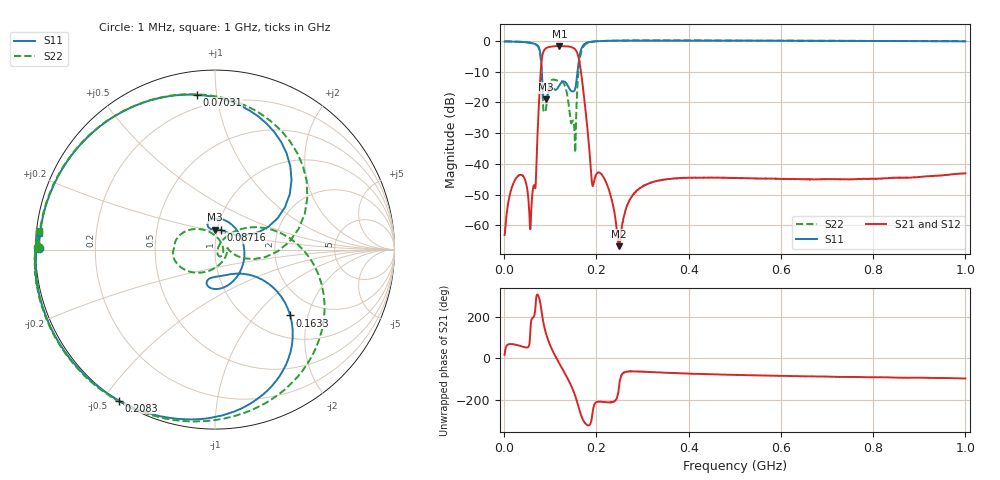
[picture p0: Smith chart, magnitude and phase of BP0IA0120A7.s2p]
!Agilent Technologies,E8358A,US41080443,A.07.50.56
!Agilent E8358A: A.07.50.56
!Date: Tuesday, October 31, 2017 22:11:44
!Correction: S11(Full 2 Port(1,2))
!S21(Full 2 Port(1,2))
!S12(Full 2 Port(1,2))
!S22(Full 2 Port(1,2))
!S2P File: Measurements: S11, S21, S12, S22:
# Hz S  dB  R 50
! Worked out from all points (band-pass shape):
!   1601 points, 1 MHz to 1 GHz, reference 50 ohm
!   highest |S21| = -1.64 dB at 119.6 MHz (marker M1); lowest = -66.7 dB at 249.5 MHz (marker M2)
!   |S21| within 3 dB of the highest: 83 MHz to 160.1 MHz (77.08 MHz wide, 63.4 % of centre)
!   lowest |S11| = -19.0 dB at 90.29 MHz (marker M3), VSWR 1.25, Z = 48.6 + j11 ohm
!   |S11| at or under -10 dB: 81.63 MHz to 159 MHz (77.38 MHz wide, 64.3 % of centre)
!   |S22| runs from -36.3 to 0.1 dB; largest |S21 - S12| = 0.004
!   S11 on the Smith chart (normalised r, x): 1 MHz: 0.01, +0.01; 70.31 MHz: 0.13, +0.88; 87.16 MHz: 1.04, +0.23; 163.3 MHz: 1.46, -1.55; 208.3 MHz: 0.00, -0.55; 1 GHz: 0.01, +0.05
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1000000  -0.17 179.4  -63.09 17.4  -62.88 18.4  -0.14 179.3
3.034562e7  -0.28 158.9  -43.90 63.0  -43.83 63.7  -0.26 158.6
5.781812e7  -0.62 127.6  -58.34 168.8  -58.27 168.5  -0.64 125.7
7.030562e7  -1.23 96.6  -38.82 -56.4  -38.80 -56.4  -1.36 90.1
7.904688e7  -4.80 42.2  -10.48 -101.3  -10.45 -100.9  -5.37 21.9
8.716375e7  -18.83 72.6  -2.96 151.5  -2.94 151.7  -23.07 4.1
9.028562e7  -19.02 90.7  -2.45 124.3  -2.43 124.4  -22.49 -51.2
1.05895e8  -15.40 62.6  -1.79 33.5  -1.76 33.5  -12.57 -171.2
1.196312e8  -14.48 -44.4  -1.64 -24.5  -1.64 -24.6  -12.88 172.6
1.364894e8  -14.17 -103.8  -1.75 -92.0  -1.77 -91.9  -17.38 123.6
1.5085e8  -16.38 -72.9  -2.38 -161.0  -2.38 -160.9  -26.57 -54.8
1.633375e8  -5.08 -41.2  -6.87 109.9  -6.90 110.0  -6.83 4.4
1.677081e8  -2.44 -58.5  -11.31 79.9  -11.35 80.2  -3.36 -26.1
1.9081e8  -0.21 -107.6  -46.48 83.6  -46.50 83.9  -0.30 -97.3
2.082925e8  -0.03 -122.4  -42.97 151.1  -42.95 151.1  -0.04 -116.6
2.495012e8  0.08 -140.4  -66.75 -130.4  -66.76 -127.5  0.11 -138.2
2.769738e8  0.10 -147.2  -50.58 -62.3  -50.57 -61.3  0.12 -146.0
3.344162e8  0.11 -156.2  -45.41 -67.4  -45.46 -67.5  0.13 -156.0
5.005e8  0.08 -168.9  -44.59 -79.6  -44.61 -79.3  0.09 -169.8
6.672081e8  0.03 -175.8  -44.95 -86.6  -45.07 -86.8  0.04 -177.0
8.339162e8  -0.04 179.2  -44.64 -91.5  -44.65 -91.5  -0.02 177.9
1e9  -0.14 174.6  -43.06 -96.7  -43.08 -96.8  -0.11 173.9
